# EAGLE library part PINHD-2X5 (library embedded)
PIN HEADER
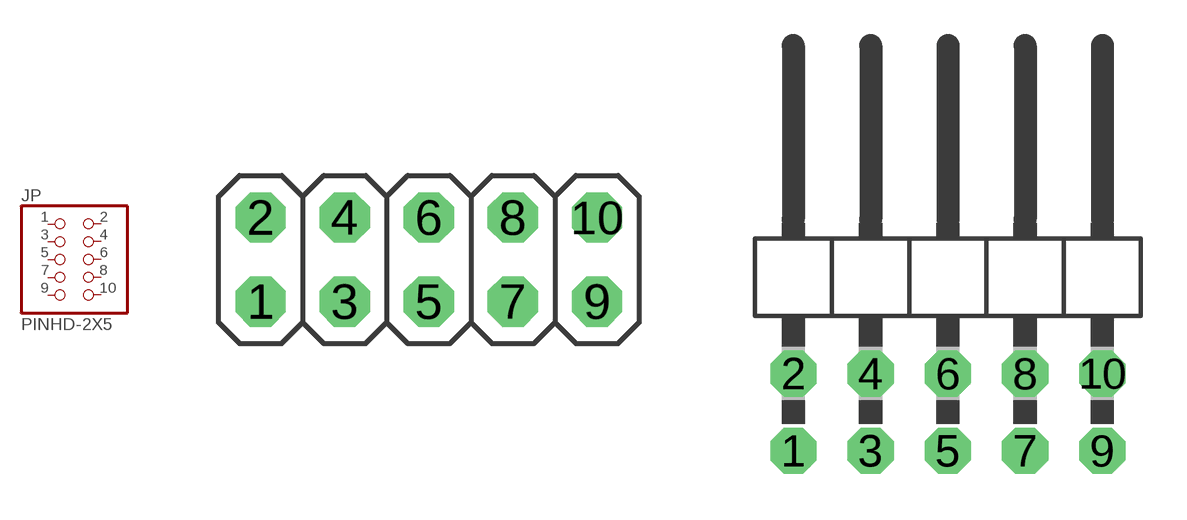
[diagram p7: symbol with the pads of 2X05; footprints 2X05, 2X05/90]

Designator prefix JP

## PINHD-2X5 (ANGLE: Straight; DESCR: Pin Header 2X5 0DEG; PACKAGE: Pin Header; PITCH: 2.54mm; POS: 10; ROWS: 2)  [2X05]
1  1  pas
2  2  pas
3  3  pas
4  4  pas
5  5  pas
6  6  pas
7  7  pas
8  8  pas
9  9  pas
10  10  pas

## PINHD-2X5/90 (ANGLE: 90; PACKAGE: Pin Header; PITCH: 2.54mm; POS: 10; ROWS: 2)  [2X05/90]
Pads as for 2X05

## PINHD-2X5/JTAG (ANGLE: Straight; DESCR: Pin Header 2X5 0DEG JTAG; PACKAGE: Pin Header; PITCH: 2.54mm; POS: 10; ROWS: 2)  [2X05/JTAG]
Pads as for 2X05

## Footprint 2X05 (pad centres in mm)
PIN HEADER
drill 1.016 octagon: 1 -5.08,-1.27; 2 -5.08,1.27; 3 -2.54,-1.27; 4 -2.54,1.27; 5 0,-1.27; 6 0,1.27; 7 2.54,-1.27; 8 2.54,1.27; 9 5.08,-1.27; 10 5.08,1.27

## Footprint 2X05/90 (pad centres in mm)
PIN HEADER
drill 1.016 octagon: 1 -5.08,-6.35; 2 -5.08,-3.81; 3 -2.54,-6.35; 4 -2.54,-3.81; 5 0,-6.35; 6 0,-3.81; 7 2.54,-6.35; 8 2.54,-3.81; 9 5.08,-6.35; 10 5.08,-3.81

## Footprint 2X05/JTAG (pad centres in mm)
PIN HEADER
drill 1 octagon: 1 -5.08,-1.27; 2 -5.08,1.27; 3 -2.54,-1.27; 4 -2.54,1.27; 5 0,-1.27; 6 0,1.27; 7 2.54,-1.27; 8 2.54,1.27; 9 5.08,-1.27; 10 5.08,1.27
